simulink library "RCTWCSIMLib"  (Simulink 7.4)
settings: Solver=ode45  SolverMode=SingleTasking  StartTime=0.0  StopTime=10.0  RelTol=1e-3
undefined symbols (not defined in the file or in its folder): L1, Maximize, Norm, wcpsi, wcsimconmask, WCSIMConstraint, WCSIMObjective, wcsimobjmask

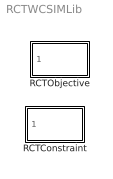
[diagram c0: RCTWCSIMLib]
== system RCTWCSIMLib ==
  RCTConstraint : Subsystem  Tag=WCSIMConstraint  StopFcn=wcsimconmask('Stop',gcb)  mask{ConType=L1 Norm, ConMfile='', ConUB=inf, ConLB=-inf, VarName=WCSIMConstraint, DataPts=inf, Decimation=1, SampleTime=-1, SaveFormat=Structure With Time, LogFixedPoint=off}
      mask prompts: ConType "Constraint Type:"; ConMfile "Constraint M-file:"; ConUB "Constraint Upper Bound:"; ConLB "Constraint Lower Bound:"; VarName "Variable name:"; DataPts "Limit data points to last:"; SampleTime "Sample time (-1 for inherited):"; SaveFormat "Save format:"; LogFixedPoint "Log fixed-point data as an fi object"
      mask init:
      | wcsimconmask('Initialize',gcb)
  RCTObjective : Subsystem  Tag=WCSIMObjective  StopFcn=wcsimobjmask('Stop',gcb)  mask{ObjType=M-file, MaxMin=Maximize, ObjMfile=wcpsi, VarName=WCSIMObjective, DataPts=inf, Decimation=1, SampleTime=-1, SaveFormat=Structure With Time, LogFixedPoint=off}
      mask prompts: ObjType "Objective Type:"; MaxMin "Max or Min:"; ObjMfile "Objective M-file:"; VarName "Variable name:"; DataPts "Limit data points to last:"; SampleTime "Sample time (-1 for inherited):"; SaveFormat "Save format:"; LogFixedPoint "Log fixed-point data as an fi object"
      mask init:
      | wcsimobjmask('Initialize',gcb)

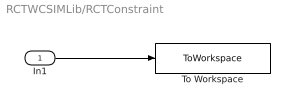
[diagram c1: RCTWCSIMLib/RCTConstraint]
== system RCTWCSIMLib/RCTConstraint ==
  In1 : Inport  OutDataType=sfix(16)  OutScaling=2^0
  To Workspace : ToWorkspace  VariableName=WCSIMConstraint  SampleTime=SampleTime  SaveFormat=Structure With Time
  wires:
  In1/1 -> To Workspace/1

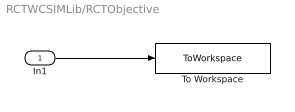
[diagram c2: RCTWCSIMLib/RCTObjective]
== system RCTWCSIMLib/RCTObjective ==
  In1 : Inport  OutDataType=sfix(16)  OutScaling=2^0
  To Workspace : ToWorkspace  VariableName=WCSIMObjective  SampleTime=SampleTime  SaveFormat=Structure With Time
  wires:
  In1/1 -> To Workspace/1
